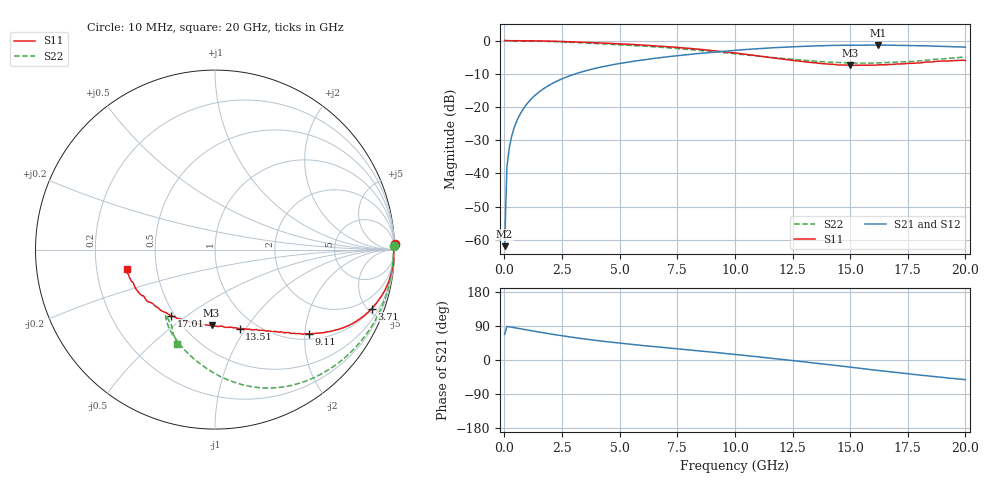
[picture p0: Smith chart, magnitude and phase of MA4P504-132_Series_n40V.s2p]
! AWR Design Environment (9226) Thu Aug 19 02:45:16 2021
! Document = 'n40V'
! nPorts: 2, nXvals: 201
# GHz S DB R 50
!Freq DBS11 AngS11 DBS21 AngS21 DBS12 AngS12 DBS22 AngS22
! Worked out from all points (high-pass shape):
!   201 points, 10 MHz to 20 GHz, reference 50 ohm
!   highest |S21| = -1.37 dB at 16.21 GHz (marker M1); lowest = -61.9 dB at 10 MHz (marker M2)
!   |S21| within 3 dB of the highest: 7.764 GHz to end of sweep
!   lowest |S11| = -7.5 dB at 15.01 GHz (marker M3), VSWR 2.46, Z = 33.8 - j34.7 ohm
!   |S11| at or under -10 dB: nowhere
!   |S22| runs from -6.8 to 0.0 dB; largest |S21 - S12| = 0.03
!   S11 on the Smith chart (normalised r, x): 10 MHz: -5, +63; 3.71 GHz: 1.04, -5.31; 9.11 GHz: 1.13, -2.09; 13.51 GHz: 0.84, -0.94; 17.01 GHz: 0.48, -0.44; 20 GHz: 0.34, -0.10
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0.01  0.02 1.8  -61.91 67.4  -60.25 67.0  -0.02 1.3
0.11  -0.04 -0.5  -38.08 88.3  -38.00 88.8  -0.06 -1.6
0.21  -0.04 -1.3  -32.39 87.7  -32.40 87.3  -0.06 -3.2
0.31  -0.03 -1.9  -29.00 86.7  -29.00 86.6  -0.06 -4.7
0.51  -0.03 -3.2  -24.67 84.4  -24.68 84.4  -0.08 -7.7
0.91  -0.05 -5.6  -19.70 80.1  -19.71 80.1  -0.11 -13.7
1.51  -0.11 -9.3  -15.46 73.6  -15.48 73.9  -0.20 -22.4
2.31  -0.25 -13.8  -12.12 65.7  -12.13 66.0  -0.38 -33.2
3.41  -0.52 -19.2  -9.34 56.1  -9.33 56.6  -0.69 -46.0
3.71  -0.60 -20.6  -8.77 53.7  -8.77 54.3  -0.79 -49.1
5.01  -1.00 -25.8  -6.90 44.6  -6.90 45.3  -1.25 -61.1
6.71  -1.66 -32.3  -5.20 34.2  -5.16 35.1  -1.98 -74.2
9.11  -3.07 -42.0  -3.48 20.1  -3.42 21.2  -3.36 -91.8
10.01  -3.74 -46.1  -2.94 14.6  -2.88 15.8  -3.97 -98.9
13.41  -6.66 -71.5  -1.64 -7.6  -1.60 -6.7  -6.18 -122.6
13.51  -6.71 -72.7  -1.62 -8.5  -1.58 -7.4  -6.23 -123.0
15.01  -7.49 -92.6  -1.41 -19.0  -1.40 -17.8  -6.74 -126.6
16.21  -7.33 -110.9  -1.37 -27.6  -1.38 -25.7  -6.74 -125.5
16.71  -7.19 -118.5  -1.40 -30.9  -1.40 -29.2  -6.60 -123.8
17.01  -7.08 -123.7  -1.42 -32.7  -1.42 -31.3  -6.48 -122.7
18.91  -6.20 -152.7  -1.70 -45.4  -1.70 -44.0  -5.55 -115.9
20  -6.00 -167.6  -1.98 -52.1  -2.01 -50.7  -4.94 -111.7
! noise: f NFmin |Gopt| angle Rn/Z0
0.01  0  1  0  2e-20
2.21  0  1  0  2e-20
4.41  0  1  0  2e-20
6.61  0  1  0  2e-20
8.81  0  1  0  2e-20
11.11  0  1  0  2e-20
13.31  0  1  0  2e-20
15.51  0  1  0  2e-20
17.71  0  1  0  2e-20
20  0  1  0  2e-20
